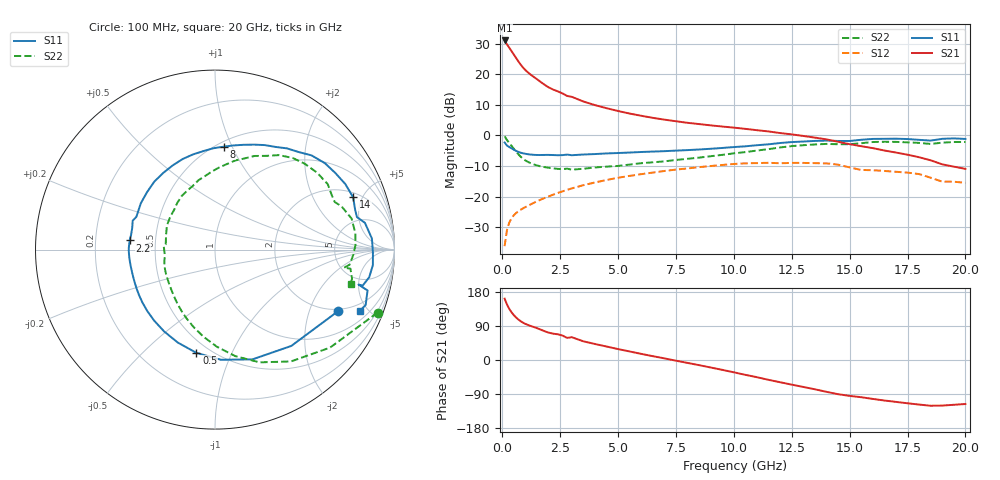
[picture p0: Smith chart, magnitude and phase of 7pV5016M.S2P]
! Infineon Technologies  Discrete & RF Semiconductors
! bfp620
! VCE = 0.50 V,  IC =  16 mA
! Common Emitter S-Parameters:  Sep 2002
# GHz  S  MA  R  50
!  f  S11  S21  S12  S22
! GHz  MAG  ANG  MAG  ANG  MAG  ANG  MAG  ANG
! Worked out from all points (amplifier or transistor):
!   59 points, 100 MHz to 20 GHz, reference 50 ohm
!   highest |S21| = 31.0 dB at 100 MHz (marker M1)
!   |S21| within 3 dB of that: start of sweep to 356 MHz
!   unconditionally stable (mu >= 1): 3.426 GHz to 10.05 GHz; 17.13 GHz to end of sweep
!   at 1 GHz: K = 0.65, MSG = 22.4 dB, |S12| = -23.4 dB
!   at 5.5 GHz: K = 1.05, MAG = 8.8 dB, |S12| = -13.2 dB
!   at 20 GHz: K = 1.64, MAG = -2.4 dB, |S12| = -15.5 dB
!   S11 on the Smith chart (normalised r, x): 100 MHz: 1.91, -3.18; 500 MHz: 0.43, -0.74; 2.2 GHz: 0.35, +0.05; 8 GHz: 0.54, +0.93; 14 GHz: 2.35, +4.23; 20 GHz: 1.52, -4.44
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0.1  0.7673 -26.5  35.62 161.9  0.0155 78.9  0.9712 -21.2
0.2  0.6847 -51.6  30.78 146.9  0.0282 64.9  0.8422 -40.4
0.3  0.6462 -71.2  27.09 135.1  0.0375 58.4  0.7533 -55.8
0.4  0.6147 -86.9  23.84 125.8  0.0444 54.0  0.6756 -68.4
0.5  0.5845 -100.2  20.9 118.2  0.0497 50.8  0.6042 -79.2
0.6  0.5579 -111.8  18.3 111.9  0.0541 48.4  0.5412 -88.9
0.7  0.5368 -121.9  16.08 106.6  0.0578 46.7  0.4887 -97.7
0.8  0.5211 -130.6  14.26 102.1  0.0612 45.6  0.4469 -105.6
1  0.5006 -143.8  11.66 95.2  0.0675 44.6  0.39 -118.5
1.2  0.4881 -153.3  10.02 90.4  0.0739 44.4  0.3554 -128.2
1.6  0.4785 -168.4  7.765 81.6  0.0872 43.8  0.3155 -145.2
2.2  0.478 173.9  5.601 69.5  0.1078 41.7  0.2898 -166.9
2.8  0.4861 160.6  4.413 58.3  0.129 38.3  0.286 176.4
3.5  0.4874 147.9  3.585 49.3  0.1538 33.2  0.285 163.1
5  0.5157 123.8  2.506 28.8  0.2034 20.4  0.3174 136.0
7  0.5528 96.6  1.811 4.3  0.2622 1.9  0.3767 108.9
8  0.5755 85.1  1.606 -7.7  0.2888 -8.1  0.4145 97.4
10.5  0.6639 59.5  1.279 -39.2  0.3499 -36.4  0.5336 72.1
13.5  0.8128 26.7  0.921 -77.3  0.3521 -71.6  0.7119 37.1
14  0.823 20.7  0.862 -84.0  0.3496 -78.6  0.7264 30.1
17  0.8839 -5.6  0.525 -110.5  0.2547 -102.8  0.7832 1.9
20  0.8757 -22.9  0.284 -116.1  0.1682 -114.6  0.7804 -14.4
